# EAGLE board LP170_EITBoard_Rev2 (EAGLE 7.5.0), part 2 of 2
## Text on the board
tNames: Level 4 V- | Level 3 V- | Level 4 V+ | Level 3 V+ | electrodes | electrodes | electrodes | electrodes | 16 | 14 | 12 | 10 | 8 | 6 | 4 | 2 | 16 | 14 | 12 | 10 | 8 | 6 | 4 | 2 | 15 | 13 | 11 | 9 | 7 | 5 | 3 | 1 | 15 | 13 | 11 | 9 | 7 | 5 | 3 | 1 | 16 | 14 | 12 | 10 | 8 | 6 | 4 | 2 | 16 | 14 | 12 | 10 | 8 | 6 | 4 | 2 | 15 | 13 | 11 | 9 | 7 | 5 | 3 | 1 | 15 | 13 | 11 | 9 | 7 | 5 | 3 | 1 | Level 4 I- | Level 3 I- | Level 4 I+ | Level 3 I+ | electrodes | electrodes | electrodes | electrodes | Level 2 V- | Level 1 V- | Level 2 V+ | Level 1 V+ | electrodes | electrodes | electrodes | electrodes | 16 | 14 | 12 | 10 | 8 | 6 | 4 | 2 | 16 | 14 | 12 | 10 | 8 | 6 | 4 | 2 | 15 | 13 | 11 | 9 | 7 | 5 | 3 | 1 | 15 | 13 | 11 | 9 | 7 | 5 | 3 | 1 | 16 | 14 | 12 | 10 | 8 | 6 | 4 | 2 | 16 | 14 | 12 | 10 | 8 | 6 | 4 | 2 | 15 | 13 | 11 | 9 | 7 | 5 | 3 | 1 | 15 | 13 | 11 | 9 | 7 | 5 | 3 | 1 | Level 2 I- | Level 1 I- | Level 2 I+ | Level 1 I+ | electrodes | electrodes | electrodes | electrodes | GND | GND | A0 | A1 | A2 | A3 | A4 | A5 | A6 | A7 | A8 | A9 | A10 | A11 | A12 | A13 | A14 | A15 | GND | IOREF | RESET | 3V3 | 5V | GND | GND | VIN | 53 | 52 | 51 | 50 | 49 | 48 | 47 | 46 | 45 | 44 | 43 | 42 | 41 | ATMEGA 2560 Board | 40 | 39 | 38 | 37 | 36 | 35 | 34 | 33 | 32 | 31 | 30 | - | + | 6 to 9V DC | 29 | 28 | 27 | 26 | LP170 - EIT-Board / DISS/ZWU 2023 / by TP | SCL | SDA | AREF | GND | 13 | 12 | 11 | 10 | 9 | 8 | 7 | 6 | 5 | 4 | 3 | 2 | TX0 | RX0 | TX3 | RX3 | TX2 | RX2 | TX1 | RX1 | SDA | SCL | 25 | 24 | USB | 23 | 22 | 5V
tDocu: BT_Status | LP171 / BT-Module | BT_TX | BT_RX | GND | 3V3 | LP171- Connected with wires and / is glued to the back of the arduino board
